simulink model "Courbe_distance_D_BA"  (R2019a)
settings: Solver=VariableStepAuto  StartTime=0.0  StopTime=6.283185307  MaxStep=0.001  RelTol=1e-6  SampleTimeConstraint=STIndependent

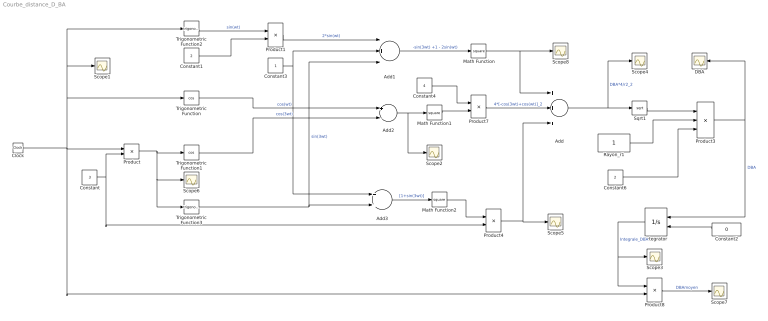
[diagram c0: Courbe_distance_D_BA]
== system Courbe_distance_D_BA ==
  Add : Sum  Inputs=+++
  Add1 : Sum  Inputs=-+-
  Add2 : Sum  Inputs=+-
  Add3 : Sum
  Clock : Clock
  Constant : Constant  Value=3
  Constant1 : Constant  Value=2
  Constant2 : Constant  Value=0
  Constant3 : Constant
  Constant4 : Constant  Value=4
  Constant6 : Constant  Value=2
  DBA : Scope
  Integrator : Integrator  InitialConditionSource=external
  Math Function : Math  Operator=square
  Math Function1 : Math  Operator=square
  Math Function2 : Math  Operator=square
  Product{,1,4,7} (4 alike) : Product
  Product3 : Product  Inputs=**/
  Product8 : Product  Inputs=*/
  Rayon_r1 : Constant
  Scope{1..8} (8 alike) : Scope
  Sqrt1 : Sqrt
  Trigonometric Function : Trigonometry  Operator=cos
  Trigonometric Function1 : Trigonometry  Operator=cos
  Trigonometric Function2 : Trigonometry
  Trigonometric Function3 : Trigonometry
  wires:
  Product/1 -> Trigonometric Function3/1, Scope6/1, Trigonometric Function1/1
  Constant/1 -> Product4/2, Product/2
  Clock/1 -> Product8/2, Trigonometric Function/1, Trigonometric Function2/1, Scope1/1, Product/1
  Trigonometric Function2/1 -> Product1/1  "sin(wt)"
  Product1/1 -> Add1/1  "2*sin(wt)"
  Add1/1 -> Math Function/1  "-sin(3wt) +1 - 2sin(wt)"
  Add2/1 -> Scope2/1, Math Function1/1
  Add3/1 -> Math Function2/1  "[1+sin(3wt)]"
  Math Function/1 -> Scope8/1, Add/1
  Add/1 -> Sqrt1/1, Scope4/1  "DBA*4/r2_2"
  Integrator/1 -> Product8/1, Scope3/1  "Integrale_DBA"
  Constant2/1 -> Integrator/2
  Product8/1 -> Scope7/1  "DBAmoyen"
  Constant1/1 -> Product1/2
  Trigonometric Function3/1 -> Add3/2, Add1/3  "sin(3wt)"
  Constant3/1 -> Add3/1, Add1/2
  Trigonometric Function1/1 -> Add2/2  "cos(3wt)"
  Trigonometric Function/1 -> Add2/1  "cos(wt)"
  Math Function1/1 -> Product7/2
  Constant4/1 -> Product7/1
  Product7/1 -> Add/2  "4*[-cos(3wt)+cos(wt)]_2"
  Sqrt1/1 -> Product3/1
  Constant6/1 -> Product3/3
  Product3/1 -> Integrator/1, DBA/1  "DBA"
  Rayon_r1/1 -> Product3/2
  Math Function2/1 -> Product4/1
  Product4/1 -> Scope5/1, Add/3
